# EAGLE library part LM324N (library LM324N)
OP Amp Quad GP 16V/32V 14-Pin PDIP Texas Instruments LM324N, Quad Op Amp, 1.2MHz, 5-28 V, 14-Pin PDIP Source: Datasheet
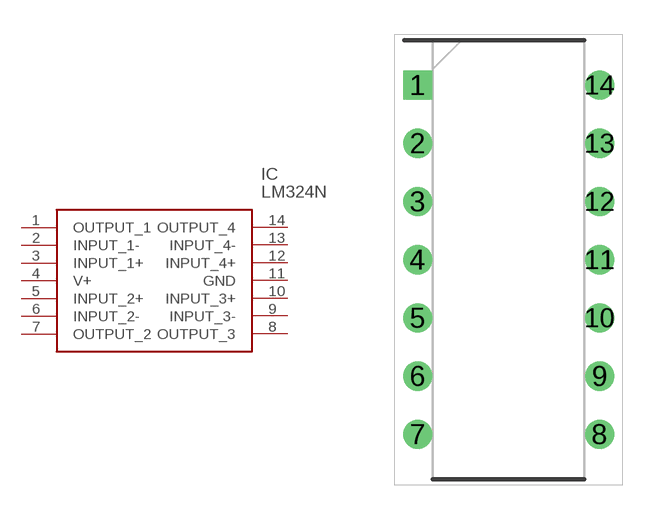
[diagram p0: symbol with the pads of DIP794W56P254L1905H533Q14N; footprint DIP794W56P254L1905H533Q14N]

Designator prefix IC

## LM324N (Description: OP Amp Quad GP 16V/32V 14-Pin PDIP Texas Instruments LM324N, Quad Op Amp, 1.2MHz, 5-28 V, 14-Pin PDIP; Height: 5.334mm; Manufacturer_Name: Texas Instruments; Manufacturer_Part_Number: LM324N; Mouser_Part_Number: 595-LM324N; Mouser_Price-Stock: https://www.mouser.co.uk/ProductDetail/Texas-Instruments/LM324N?qs=VolsR0DjNPqtt3qB38bTqw%3D%3D)  [DIP794W56P254L1905H533Q14N]
1  OUTPUT_1
2  INPUT_1-
3  INPUT_1+
4  V+
5  INPUT_2+
6  INPUT_2-
7  OUTPUT_2
8  OUTPUT_3
9  INPUT_3-
10  INPUT_3+
11  GND
12  INPUT_4+
13  INPUT_4-
14  OUTPUT_4

## Footprint DIP794W56P254L1905H533Q14N (pad centres in mm)
NFF0014A
drill 0.759 pad 1.159 square: 1 -3.969,7.62
drill 0.759 pad 1.159: 2 -3.969,5.08; 3 -3.969,2.54; 4 -3.969,0; 5 -3.969,-2.54; 6 -3.969,-5.08; 7 -3.969,-7.62; 8 3.969,-7.62; 9 3.969,-5.08; 10 3.969,-2.54; 11 3.969,0; 12 3.969,2.54; 13 3.969,5.08; 14 3.969,7.62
